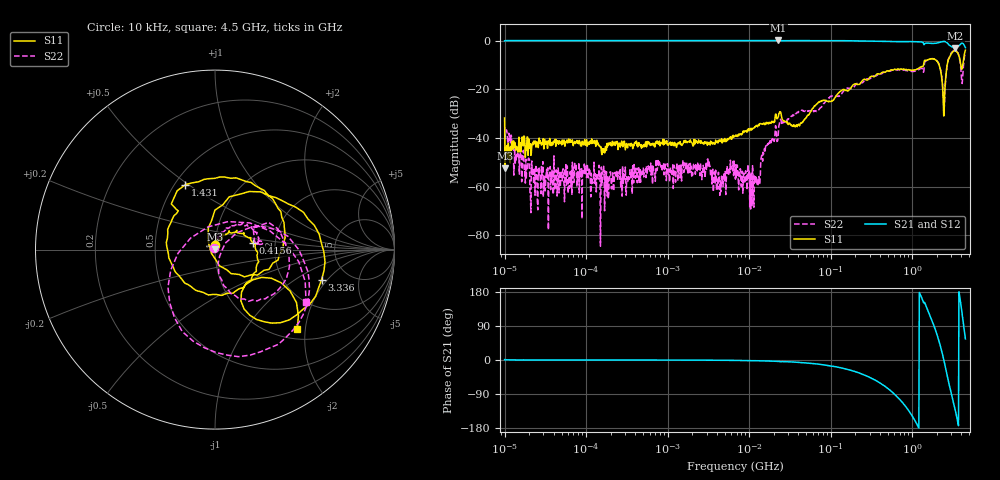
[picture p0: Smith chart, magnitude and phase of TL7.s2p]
!Siglent Technologies,SNA5004A,SNA5XCED5R0097,V1.0.0.2.10.R9
!Date: 2024-11-24 16:59:56
!Data & Calibration Information:
!Freq	S11:F2(ON)	S21:F2(ON)	S12:F2(ON)	S22:F2(ON)
# Hz S DB R 50
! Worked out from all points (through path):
!   1001 points, 10 kHz to 4.5 GHz, reference 50 ohm
!   highest |S21| = 0.11 dB at 22.8 MHz (marker M1); lowest = -3.0 dB at 3.379 GHz (marker M2)
!   group delay of S21, straight-line fit = 407 ps
!   lowest |S11| = -52.4 dB at 10.13 kHz (marker M3), VSWR 1.00, Z = 50.1 + j0.198 ohm
!   |S11| at or under -10 dB: start of sweep to 1.38 GHz; 2.148 GHz to 2.685 GHz (537.3 MHz wide, 22.2 % of centre); 3.955 GHz to 4.178 GHz (223 MHz wide, 5.48 % of centre)
!   |S22| runs from -84.4 to -3.9 dB; largest |S21 - S12| = 0.024
!   S11 on the Smith chart (normalised r, x): 10 kHz: 1.00, +0.05; 415.6 MHz: 1.53, +0.12; 1.431 GHz: 0.57, +0.49; 3.336 GHz: 3.21, -1.74; 4.5 GHz: 1.21, -1.81
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10000  -31.75 86.9  -0.03 0.8  -0.03 0.9  -40.13 134.8
10131.02  -52.38 55.1  0.02 0.3  -0.04 0.2  -40.38 111.1
23920.22  -42.28 3.8  0.06 0.1  -0.00 -0.0  -56.28 116.1
87919.76  -43.33 10.4  0.06 0.0  0.00 -0.1  -52.56 -52.6
772988.4  -42.57 19.6  0.06 -0.1  0.01 -0.2  -51.27 -35.6
3112194  -42.09 30.7  0.07 -0.5  0.01 -0.7  -48.57 -47.5
4253474  -41.41 45.0  0.06 -0.7  -0.01 -0.8  -57.40 -146.0
6708204  -39.20 68.9  0.05 -1.0  -0.02 -1.2  -55.08 -176.6
1.205038e7  -35.11 81.6  0.06 -1.9  -0.02 -2.0  -55.92 131.3
2.280385e7  -31.31 106.7  0.11 -3.8  0.04 -3.7  -37.82 88.0
5.897837e7  -28.31 64.6  0.02 -9.2  -0.05 -9.2  -28.84 90.3
4.155991e8  -13.34 9.8  -0.24 -62.3  -0.31 -62.1  -13.64 41.4
5.185364e8  -12.54 -7.7  -0.32 -77.3  -0.37 -77.0  -12.45 31.7
8.842213e8  -12.04 -92.6  -0.36 -130.2  -0.42 -130.0  -12.38 9.1
1.431297e9  -8.02 114.5  -1.22 150.4  -1.27 150.8  -8.69 18.6
1.930873e9  -7.83 18.1  -1.05 79.2  -1.13 79.7  -7.72 -36.8
2.409119e9  -24.84 -85.8  -0.30 6.4  -0.37 7.0  -22.36 -76.6
2.816416e9  -7.47 45.4  -1.64 -61.1  -1.68 -60.4  -7.18 5.0
3.335713e9  -4.19 -15.7  -2.94 -127.3  -3.01 -126.6  -3.95 -56.2
3.379417e9  -4.22 -20.2  -2.95 -132.6  -3.03 -132.0  -4.06 -61.0
3.849231e9  -7.67 -62.1  -1.67 165.1  -1.73 165.8  -8.17 -130.2
4.5e9  -3.90 -44.1  -2.84 55.7  -2.91 57.0  -4.68 -29.7
